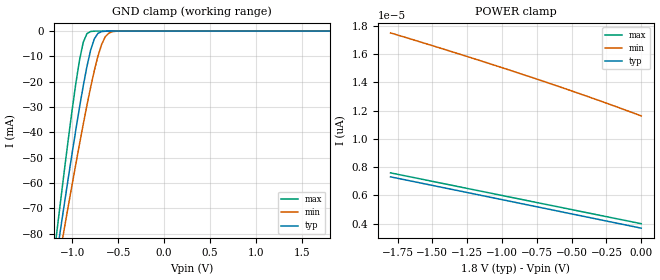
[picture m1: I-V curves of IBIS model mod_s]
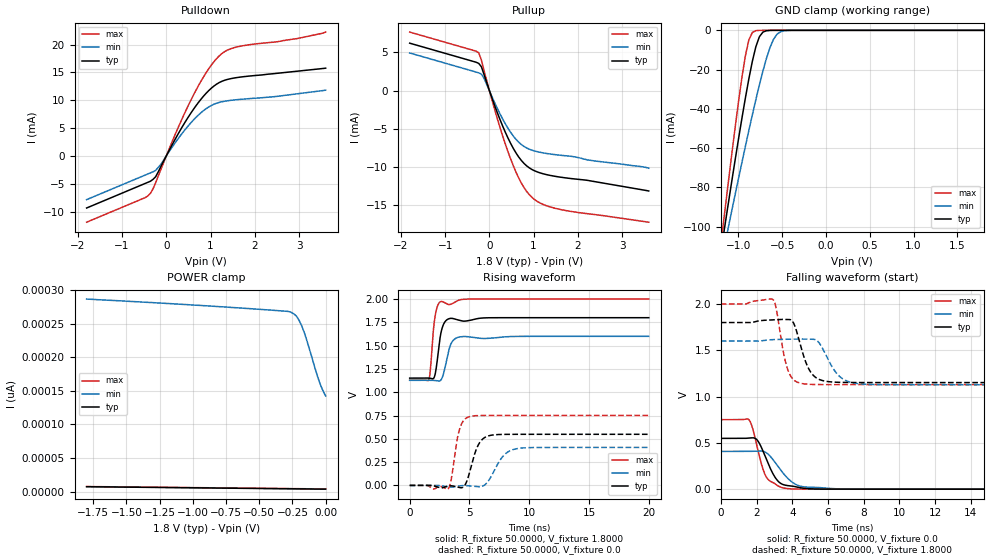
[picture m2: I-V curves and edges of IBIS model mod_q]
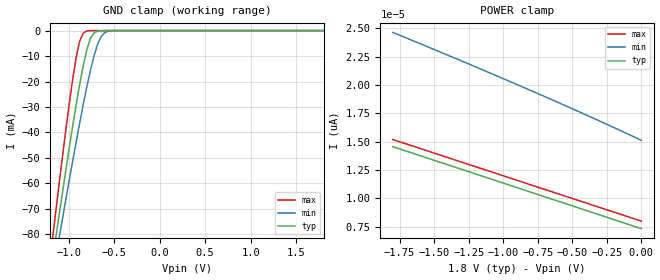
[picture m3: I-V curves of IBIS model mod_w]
| IBIS (I/O, Buffer, Information, Specification) Model, officially
| electronic behavioral standard for Buffer structures of digital pins.
[IBIS ver]  4.0
[File name] m95m02ef_1v8_dfn8.ibs
[File Rev]  1.0
[Source]   CAD & Design Services (Catania) - STMicroelectronics
[Date]   21 Jan 2026
[Notes]
   (Note1)  This IBIS model includes DFN8 Package parasitic data
   (Note2)  This IBIS model considers: VCC=1.80(TYP), 1.60(MIN), 2.00(MAX)
   (Note3)  This IBIS model has some Notes about the non-monotonicity
   of the I-V curves, but they are not indicative of problems
   inside the model;
[Disclaimer]
   Customers are solely responsible for all aspects of their
   own product designs or applications using this IBIS Model.
   STMicroelectronics assumes no liability for Custmer Designs
   and applications associated to this IBIS Model.
   In the use of this IBIS Model Customer shall not modify,
   disassemble, alter this Model in whole or in part.
   If Customers do not accept these terms, the IBIS Model
   may not be used. For any problems or modifications please
   contact STMicroelectronics (www.st.com).
[Copyright] (c) 2026 STMicroelectronics
|   Component M95M02EF
[Component] M95M02EF
[Manufacturer] STMicroelectronics
[Package]
| variable   typ   min   max
R_pkg   0.0   0.0   0.0
L_pkg   0.0H   0.0H   0.0H
C_pkg   0.0F   0.0F   0.0F
[Pin]  signal_name   model_name   R_pin   L_pin   C_pin
1   SN   mod_s   0.0   0.0   0.0
2   Q   mod_q   0.0   0.0   0.0
3   WN   mod_w   0.0   0.0   0.0
4   GND   GND   0.0   0.0   0.0
5   D   mod_d   0.0   0.0   0.0
6   C   mod_c   0.0   0.0   0.0
7   H   mod_h   0.0   0.0   0.0
8   VCC   POWER   0.0   0.0   0.0
[Package Model]  182694_DFN8   | also called 182694_MLP_2x3
[Define Package Model]  182694_DFN8
[Manufacturer]  STMicroelectronics
[OEM]  STMicroelectronics
[Description]  8 pin MLP 2x3
[Number Of Pins]  8
[Pin Numbers]
|Pin Num   Terminal Name
1   | net1
2   | net2
3   | net3
4   | net4_GND
5   | net5
6   | net6
7   | net7
8   | net8_VDD
[Model Data]
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[End Model Data]
[End Package Model]
| Models and submodels in the file (6): mod_s (Input), mod_q (I/O), mod_w (Input), mod_d (Input), mod_c (Input), mod_h (Input)
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|   Model mod_s
[Model]   mod_s
Model_type Input
Vinl   =   0.540V
Vinh   =   1.260V
C_comp   3.207pF   3.064pF   3.356pF
[Temperature Range]  25.0000   85.0000   -40.0000
[Voltage Range]   1.8000V   1.6000V   2.0000V
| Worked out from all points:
|   GND clamp passes 1 mA (typ) near -0.72 V on its own axis
[GND_clamp]
|Voltage   I(typ)   I(min)   I(max)
-1.8V     -248.6mA   -231.3mA   -277.7mA
-1.16V    -86.35mA   -93.41mA   -77.15mA
-1.12V    -76.58mA   -85.05mA   -65.2mA
-1.08V    -66.91mA   -76.75mA   -53.44mA
-1V       -48mA      -60.39mA   -30.91mA
-920mV    -30.02mA   -44.49mA   -11.36mA
-880mV    -21.65mA   -36.8mA    -4.45mA
-840mV    -14.02mA   -29.36mA   -1.025mA
-760mV    -3.101mA   -15.69mA   -22.27uA
-680mV    -210.8uA   -5.26mA    -416.9nA
-560mV    -2.037uA   -222.4uA   -1.075nA
1.8V      3.684pA    12.36pA    3.6pA
[POWER_clamp]
|Voltage   I(typ)   I(min)   I(max)
-1.8V     7.317pA    17.51pA    7.6pA
-1.26V    6.229pA    15.87pA    6.52pA
-800mV    5.301pA    14.4pA     5.6pA
-380mV    4.453pA    12.99pA    4.76pA
0V        3.684pA    11.63pA    4pA
|   Model mod_q
[Model]   mod_q
Model_type I/O
Polarity   Non-Inverting
Enable   Active-Low
Vinl   =   0.540V
Vinh   =   1.260V
Vmeas  =   0.900V
Cref   =   30pF
C_comp   4.038pF   3.859pF   4.226pF
[Temperature Range]  25.0000   85.0000   -40.0000
[Voltage Range]   1.8000V   1.6000V   2.0000V
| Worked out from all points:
|   slope of the pulldown table from 0 to 0.27 V, typ, clamps not added: 67.8 ohm
|   slope of the pullup table from 0 to 0.27 V, typ, clamps not added: 63.9 ohm
|   GND clamp passes 1 mA (typ) near -0.72 V on its own axis
|   rising waveform, R_fixture 50.0000, V_fixture 1.8000: 20-80 % time 433ps typ, 530ps min, 366ps max; typ from 1.15 V to 1.8 V
|   rising waveform, R_fixture 50.0000, V_fixture 0.0: 20-80 % time 814ps typ, 1.15ns min, 584ps max; typ from 0 V to 0.548 V
|   falling waveform, R_fixture 50.0000, V_fixture 0.0: 20-80 % time 803ps typ, 1.06ns min, 637ps max; typ from 0.548 V to 0 V
|   falling waveform, R_fixture 50.0000, V_fixture 1.8000: 20-80 % time 680ps typ, 891ps min, 511ps max; typ from 1.8 V to 1.15 V
[Pulldown]   | MIN new
|Voltage   I(typ)   I(min)   I(max)
-1.8V     -9.354mA   -7.852mA   -11.9mA
-480mV    -4.954mA   -3.452mA   -7.503mA
-360mV    -4.554mA   -3.052mA   -6.733mA
-240mV    -3.743mA   -2.603mA   -4.809mA
-120mV    -1.883mA   -1.497mA   -2.386mA
240mV     3.562mA    2.793mA    4.573mA
600mV     8.216mA    6.336mA    10.71mA
960mV     11.74mA    8.802mA    15.67mA
1.26V     13.42mA    9.736mA    18.41mA
1.68V     14.17mA    10.17mA    19.72mA
2.94V     15.2mA     11.14mA    21.06mA
3.6V      15.77mA    11.82mA    22.25mA
[Pullup]   | MIN new
|Voltage   I(typ)   I(min)   I(max)
-1.8V     6.212mA    4.924mA    7.664mA
-240mV    3.558mA    2.316mA    4.944mA
-180mV    3.117mA    2.153mA    3.995mA
-120mV    2.102mA    1.612mA    2.634mA
180mV     -2.906mA   -2.346mA   -3.692mA
480mV     -6.924mA   -5.479mA   -8.962mA
660mV     -8.691mA   -6.758mA   -11.42mA
780mV     -9.54mA    -7.321mA   -12.69mA
1.02V     -10.52mA   -7.924mA   -14.29mA
1.26V     -10.98mA   -8.221mA   -15.04mA
1.62V     -11.37mA   -8.493mA   -15.62mA
3.6V      -13.17mA   -10.18mA   -17.26mA
[GND_clamp]
|Voltage   I(typ)   I(min)   I(max)
-1.8V     -294.1mA   -253.2mA   -343.6mA
-1.2V     -113.1mA   -119mA     -109.3mA
-1.16V    -101.4mA   -110.3mA   -94.31mA
-1.12V    -89.76mA   -101.6mA   -79.46mA
-1.08V    -78.28mA   -92.93mA   -64.88mA
-920mV    -34.54mA   -59.15mA   -13.02mA
-840mV    -15.73mA   -43.01mA   -1.053mA
-760mV    -3.267mA   -27.8mA    -22.28uA
-720mV    -920.4uA   -20.79mA   -3.05uA
-600mV    -9.651uA   -4.685mA   -7.81nA
-520mV    -429.6nA   -743.9uA   -150.4pA
1.8V      3.684pA    266.8pA    3.6pA
[POWER_clamp]
|Voltage   I(typ)   I(min)   I(max)
-1.8V     7.317pA    286.4pA    7.6pA
-740mV    5.18pA     274.4pA    5.48pA
-280mV    4.251pA    268pA      4.56pA
-260mV    4.21pA     266.7pA    4.52pA
-220mV    4.129pA    261.1pA    4.44pA
-200mV    4.089pA    254.8pA    4.4pA
-180mV    4.048pA    246.5pA    4.36pA
-160mV    4.008pA    236.2pA    4.32pA
-140mV    3.967pA    223.9pA    4.28pA
-60mV     3.806pA    170.7pA    4.12pA
-40mV     3.765pA    159.3pA    4.08pA
0V        3.684pA    142.2pA    4pA
[Ramp]
| variable   typ   min   max
dV/dt_r   0.3290/0.9015n   0.2446/1.2464n   0.4506/0.5869n
dV/dt_f   0.3891/0.7342n   0.2835/0.9280n   0.5227/0.5584n
R_load = 50.0000
[Rising Waveform]
R_fixture= 50.0000
V_fixture= 1.8000
V_fixture_min= 1.6000
V_fixture_max= 2.0000
|time   V(typ)   V(min)   V(max)
0s        1.151V     1.128V     1.129V
1.62ns    1.151V     1.129V     1.14V
1.74ns    1.149V     1.128V     1.252V
1.98ns    1.147V     1.127V     1.662V
2.1ns     1.178V     1.126V     1.794V
2.58ns    1.614V     1.127V     1.973V
2.9ns     1.746V     1.233V     1.963V
3.42ns    1.793V     1.51V      1.944V
4.1ns     1.774V     1.591V     1.988V
20ns      1.8V       1.6V       2V
[Rising Waveform]
R_fixture= 50.0000
V_fixture= 0.0
V_fixture_min= 0.0
V_fixture_max= 0.0
|time   V(typ)   V(min)   V(max)
0s        2.885nV    172.8nV    1.863nV
3.26ns    -6.221mV   -15.84mV   -31.9mV
4.14ns    -22.05mV   -5.781mV   588.8mV
4.6ns     -1.709mV   -1.848mV   708.9mV
5.02ns    143.8mV    -5.242mV   738.9mV
5.74ns    434.4mV    -15.06mV   749.5mV
6.7ns     535.5mV    70.27mV    750.8mV
7.78ns    547.4mV    308.9mV    750.8mV
8.98ns    548.4mV    394.5mV    750.8mV
20ns      548.5mV    407.6mV    750.8mV
[Falling Waveform]
R_fixture= 50.0000
V_fixture= 0.0
V_fixture_min= 0.0
V_fixture_max= 0.0
|time   V(typ)   V(min)   V(max)
0s        548.5mV    407.6mV    750.8mV
1.58ns    551.7mV    408mV      748.7mV
1.78ns    555mV      409.3mV    657mV
2.02ns    533.9mV    411.4mV    469.6mV
2.5ns     346.9mV    398.8mV    148.1mV
3.06ns    121.6mV    283.4mV    54.55mV
3.58ns    44.25mV    152mV      10.2mV
4.46ns    14.91mV    32.03mV    480uV
6.38ns    105.5uV    4.92mV     2.446uV
20ns      1.553nV    162nV      2.439nV
[Falling Waveform]
R_fixture= 50.0000
V_fixture= 1.8000
V_fixture_min= 1.6000
V_fixture_max= 2.0000
|time   V(typ)   V(min)   V(max)
0s        1.8V       1.6V       2V
2.96ns    1.829V     1.616V     2.041V
3.72ns    1.833V     1.62V      1.306V
4.08ns    1.792V     1.621V     1.181V
4.48ns    1.541V     1.622V     1.143V
4.88ns    1.316V     1.621V     1.133V
5.36ns    1.2V       1.608V     1.13V
6.56ns    1.154V     1.235V     1.129V
7.52ns    1.152V     1.144V     1.129V
20ns      1.151V     1.128V     1.129V
|   Model mod_w
[Model]   mod_w
Model_type Input
Vinl   =   0.540V
Vinh   =   1.260V
C_comp   3.207pF   3.064pF   3.356pF
[Temperature Range]  25.0000   85.0000   -40.0000
[Voltage Range]   1.8000V   1.6000V   2.0000V
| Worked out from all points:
|   GND clamp passes 1 mA (typ) near -0.72 V on its own axis
[GND_clamp]
|Voltage   I(typ)   I(min)   I(max)
-1.8V     -248.6mA   -231.3mA   -277.7mA
-1.16V    -86.36mA   -93.41mA   -77.15mA
-1.12V    -76.58mA   -85.05mA   -65.2mA
-1.08V    -66.91mA   -76.75mA   -53.44mA
-1V       -48mA      -60.39mA   -30.92mA
-920mV    -30.02mA   -44.49mA   -11.36mA
-880mV    -21.65mA   -36.8mA    -4.455mA
-840mV    -14.02mA   -29.36mA   -1.03mA
-760mV    -3.105mA   -15.69mA   -23.76uA
-680mV    -212.7uA   -5.263mA   -482.6nA
-560mV    -2.094uA   -223.5uA   -1.252nA
1.8V      7.336pA    16.26pA    7.2pA
[POWER_clamp]
|Voltage   I(typ)   I(min)   I(max)
-1.8V     14.57pA    24.64pA    15.2pA
-1.24V    12.32pA    21.81pA    12.96pA
-780mV    10.47pA    19.41pA    11.12pA
-380mV    8.865pA    17.26pA    9.52pA
0V        7.336pA    15.13pA    8pA
